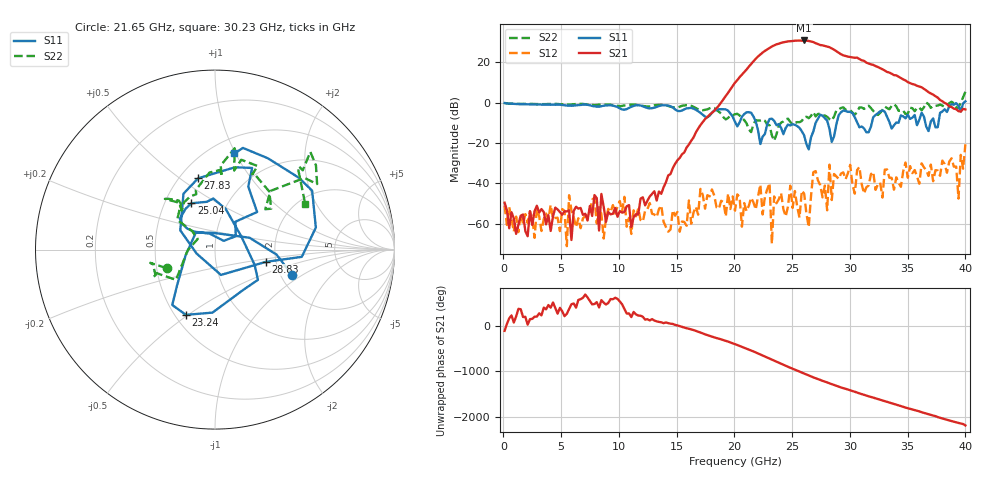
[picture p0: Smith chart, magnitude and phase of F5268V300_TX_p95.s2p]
!S2P File: Measurements: S11,S21,S12,S22
# MHz S  RI  R 50
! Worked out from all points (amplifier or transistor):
!   201 points, 100 MHz to 40 GHz, reference 50 ohm
!   highest |S21| = 30.8 dB at 26.04 GHz (marker M1)
!   |S21| within 3 dB of that: 23.24 GHz to 28.02 GHz (4.78 GHz wide, 18.7 % of centre)
!   unconditionally stable (mu >= 1): start of sweep to 26.81 GHz; 30.85 GHz to 32.98 GHz; 33.11 GHz to 36.57 GHz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
!   at 6.684 GHz: K = 9312.29, MAG = -37.7 dB, |S12| = -62.3 dB
!   at 20.05 GHz: K = 50.74, MAG = 11.7 dB, |S12| = -53.6 dB
!   at 40 GHz: K = 2.36, MSG = 8.6 dB, |S12| = -20.7 dB
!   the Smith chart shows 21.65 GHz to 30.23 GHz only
!   S11 on the Smith chart (normalised r, x): 21.65 GHz: 2.30, -0.81; 23.24 GHz: 0.57, -0.49; 25.04 GHz: 0.68, +0.38; 27.83 GHz: 0.62, +0.59; 28.83 GHz: 1.76, -0.26; 30.23 GHz: 0.65, +0.99
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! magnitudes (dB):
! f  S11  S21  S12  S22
! 100 MHz  -0.2  -49.6  -51.1  -0.2
! 5.088 GHz  -1.2  -55.6  -52.8  -0.8
! 5.487 GHz  -1.5  -54.0  -71.2  -0.9
! 5.686 GHz  -1.5  -53.5  -46.0  -1.0
! 6.883 GHz  -1.0  -55.7  -57.4  -0.7
! 13.47 GHz  -1.7  -44.1  -52.8  -1.1
! 20.05 GHz  -9.5  9.9  -53.6  -5.8
! 21.65 GHz  -6.9  20.4  -49.5  -10.8
! 23.04 GHz  -8.2  27.0  -40.0  -11.2
! 23.24 GHz  -8.0  27.8  -70.0  -16.3
! 23.44 GHz  -9.1  28.4  -46.6  -18.9
! 25.04 GHz  -10.8  30.5  -52.3  -10.9
! 26.04 GHz  -16.3  30.8  -45.1  -7.3
! 26.43 GHz  -23.2  30.5  -61.8  -7.8
! 26.83 GHz  -14.3  30.0  -34.6  -4.8
! 27.83 GHz  -7.8  28.1  -41.2  -6.4
! 28.83 GHz  -10.7  25.5  -36.7  -3.9
! 30.23 GHz  -5.2  22.4  -40.8  -5.0
! 33.42 GHz  -9.6  14.8  -37.3  -3.3
! 38.8 GHz  -0.8  -2.2  -27.7  0.4
! 39.4 GHz  -1.7  -4.3  -47.6  -2.7
! 40 GHz  0.6  -3.4  -20.7  5.3
